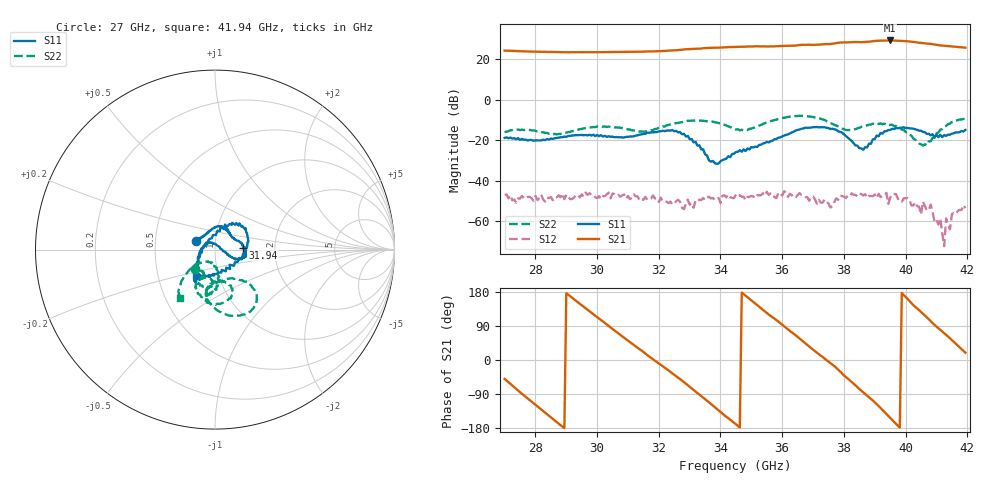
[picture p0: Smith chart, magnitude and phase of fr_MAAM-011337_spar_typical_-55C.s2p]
! Created Thu Jan 25 15:57:56 2024
# hz S db R 50
! 2 Port Network Data from SP1.SP block
! freq  dbS11  angS11  dbS21  angS21  dbS12  angS12  dbS22  angS22
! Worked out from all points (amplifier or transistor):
!   240 points, 27 GHz to 41.94 GHz, reference 50 ohm
!   highest |S21| = 29.1 dB at 39.5 GHz (marker M1)
!   |S21| within 3 dB of that: 34.87 GHz to 41.55 GHz (6.681 GHz wide, 17.5 % of centre)
!   unconditionally stable (mu >= 1): start of sweep to end of sweep
!   at 29.5 GHz: K = 7.01, MAG = 23.5 dB, |S12| = -46.7 dB
!   at 34.5 GHz: K = 5.37, MAG = 26.1 dB, |S12| = -46.8 dB
!   at 41.94 GHz: K = 10.77, MAG = 26.2 dB, |S12| = -53.5 dB
!   S11 on the Smith chart (normalised r, x): 27 GHz: 0.81, +0.08; 31.94 GHz: 1.37, +0.03; 41.94 GHz: 0.78, -0.23
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2.70046e10  -18.89 156.1  24.08 -49.9  -46.96 -112.6  -16.17 -136.2
2.762948e10  -19.86 139.4  23.71 -93.4  -48.57 -135.2  -15.04 -120.3
2.844181e10  -19.71 109.9  23.45 -147.2  -48.57 -159.8  -16.88 -116.1
2.95041e10  -17.46 72.7  23.28 144.6  -46.67 173.1  -14.48 -125.4
3.062888e10  -18.46 43.9  23.38 73.9  -47.40 128.3  -13.69 -95.2
3.194111e10  -16.03 4.0  23.75 -5.6  -48.72 82.6  -14.40 -117.8
3.20036e10  -15.68 5.3  23.79 -9.2  -50.44 78.6  -13.86 -117.5
3.275345e10  -17.09 -20.0  24.56 -54.1  -53.29 72.8  -11.15 -103.9
3.344081e10  -24.52 -11.9  25.26 -99.0  -48.49 52.7  -10.46 -81.5
3.45031e10  -25.84 125.9  25.91 -169.5  -46.77 29.0  -14.75 -74.0
3.512798e10  -23.21 174.0  26.21 148.9  -48.53 11.8  -13.72 -99.9
3.587782e10  -18.81 -143.6  26.30 101.3  -45.89 -17.5  -9.49 -88.7
3.65027e10  -14.96 -123.6  26.73 60.8  -46.94 -35.2  -8.11 -67.4
3.70026e10  -13.58 -121.3  26.98 27.5  -47.74 -59.9  -8.62 -51.5
3.781494e10  -15.65 -132.2  27.92 -25.5  -49.37 -32.5  -13.25 -51.4
3.843981e10  -22.73 172.7  28.27 -71.8  -47.69 -71.6  -14.19 -93.0
3.90022e10  -19.45 75.4  28.83 -111.7  -46.74 -92.2  -12.02 -101.7
3.95021e10  -14.99 50.7  29.09 -152.8  -48.39 -116.6  -12.61 -93.5
4.0002e10  -14.01 28.9  28.75 166.3  -48.53 -144.8  -15.96 -84.3
4.068936e10  -16.90 -19.2  27.59 112.7  -54.63 161.9  -22.49 -120.1
4.125175e10  -17.52 -74.9  26.53 70.9  -72.20 -62.6  -13.39 -139.6
4.193911e10  -14.98 -125.9  25.55 19.1  -53.47 -63.6  -9.51 -126.1
